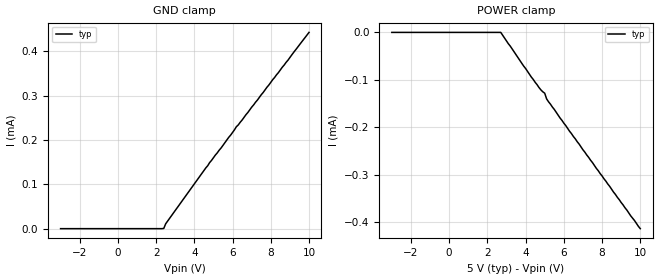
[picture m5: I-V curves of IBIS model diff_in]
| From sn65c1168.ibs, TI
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|   diff_in Model
[Model]   diff_in
Model_type   Input
Vinl = 0.8
Vinh = 2
|   typ   min   max
C_comp   123pF   NA   NA
| Where Nom  PVT is Nominal Process, 5.0V, 27C
[Voltage Range]   5   NA   NA
|Junction Temperature
[Temperature Range]   27   NA   NA
[Power Clamp Reference]   5   NA   NA
[GND Clamp Reference]   0   NA   NA
[GND Clamp]
|   Voltage   I(typ)   I(min)   I(max)
-3V       0A         NA         NA
2.4V      500nA      NA         NA
2.5V      11uA       NA         NA
4.8V      149uA      NA         NA
5.4V      182uA      NA         NA
6.2V      230uA      NA         NA
6.5V      245uA      NA         NA
10V       442.6uA    NA         NA
[POWER Clamp]
|   Voltage   I(typ)   I(min)   I(max)
-3V       0A         NA         NA
2.7V      0A         NA         NA
4.3V      -94uA      NA         NA
4.8V      -121uA     NA         NA
5V        -128uA     NA         NA
5.1V      -140uA     NA         NA
5.8V      -180uA     NA         NA
10V       -413uA     NA         NA
